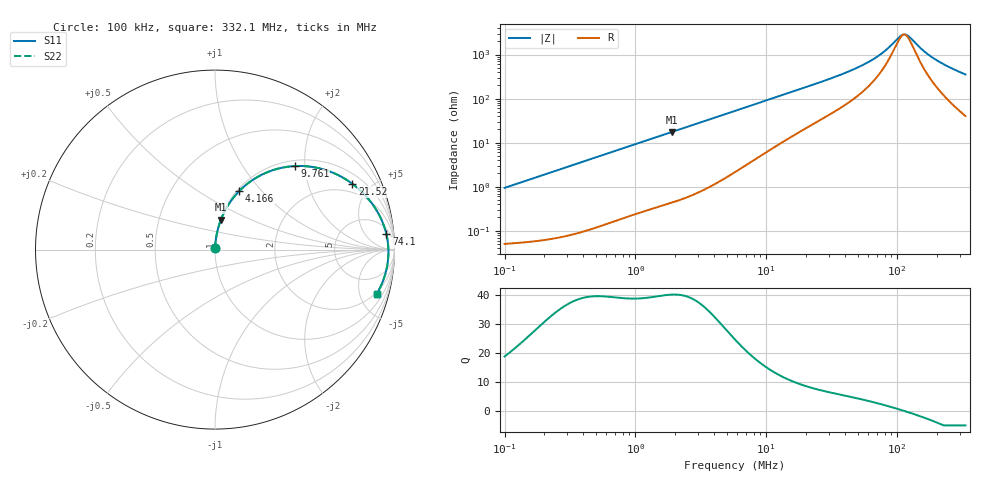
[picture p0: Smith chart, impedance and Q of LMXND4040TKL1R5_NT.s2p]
! LMXND4040TKL1R5_NT  S-PARAMETER MODEL  ( Standard Model )
! Model Generated by TAIYO YUDEN Corporation (https://www.yuden.co.jp/en/)
! Version 1.0
! TAIYO YUDEN Control No. 20251120
! Copyright(c) 2025 TAIYO YUDEN CO.,LTD. All Rights Reserved.
! Product Description (link to TY-COMPAS)
! https://ds.yuden.co.jp/TYCOMPAS/or/detail?pn=LMXND4040TKL1R5NNT&u=M
! Products Name : Inductors
! Characteristics :
!  Inductance : 1.5 [uH] , SRF(min) : 75 [MHz] , DC Resistance(max) : 0.045 [Ohm]
!  Rated Current : Saturation  3300 [mA] , Temp Rise  3100 [mA] (40 [degC])
!  Case Size : 4.0 x 4.0 / 0.157 x 0.157 [mm/inch] , Thickness : 1.8 / 0.071 [mm/inch]
!  (Conditions: Temperature = 25 [degC] , DC Bias Current = 0 [A])
! External Node Assignments :
!  1  o---GGG---o  2
! GND o---------o GND
! Frequency Range : 0.1MHz  -  332.076389MHz  [ 402 STEP ]
# MHz S RI R 50
! Freq[MHz].  S11 Real  S11 Imag  S21 Real  S21 Imag  S12 Real  S12 Imag  S22 Real  S22 Imag
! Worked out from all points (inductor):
!   401 points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, 100 kHz to 332.1 MHz, reference 50 ohm
!   read as one part in series: L = 1.49 uH near 104.1 kHz
!   highest Q = 40 at 1.89 MHz (marker M1), where L = 1.45 uH
!   self-resonance near 113 MHz
!   S11 on the Smith chart (normalised r, x): 100 kHz: 1.00, +0.02; 4.166 MHz: 1.02, +0.76; 9.761 MHz: 1.12, +1.77; 21.52 MHz: 1.48, +3.88; 74.1 MHz: 9, +18; 332.1 MHz: 1.80, -7.02
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0.1  0.00059 0.00939  0.9994 -0.00939  0.9994 -0.00939  0.00059 0.00939
0.388873  0.00224 0.0361  0.9978 -0.0361  0.9978 -0.0361  0.00224 0.0361
1.512219  0.0221 0.1349  0.9779 -0.1349  0.9779 -0.1349  0.0221 0.1349
1.889943  0.0329 0.1662  0.9671 -0.1662  0.9671 -0.1662  0.0329 0.1662
4.166482  0.1339 0.325  0.8661 -0.325  0.8661 -0.325  0.1339 0.325
5.762607  0.2257 0.3981  0.7743 -0.3981  0.7743 -0.3981  0.2257 0.3981
9.761116  0.4449 0.4654  0.5551 -0.4654  0.5551 -0.4654  0.4449 0.4654
14.05902  0.6102 0.4451  0.3898 -0.4451  0.3898 -0.4451  0.6102 0.4451
21.51891  0.766 0.3661  0.234 -0.3661  0.234 -0.3661  0.766 0.3661
22.4092  0.7779 0.357  0.2221 -0.357  0.2221 -0.357  0.7779 0.357
45.55486  0.9162 0.1902  0.0838 -0.1902  0.0838 -0.1902  0.9162 0.1902
59.28911  0.9415 0.1321  0.0585 -0.1321  0.0585 -0.1321  0.9415 0.1321
74.09842  0.9552 0.0852  0.0448 -0.0852  0.0448 -0.0852  0.9552 0.0852
87.14324  0.9615 0.0521  0.0385 -0.0521  0.0385 -0.0521  0.9615 0.0521
106.7246  0.9657 0.0115  0.0343 -0.0115  0.0343 -0.0115  0.9657 0.0115
113.4159  0.9662 -0.00073  0.0338 0.00073  0.0338 0.00073  0.9662 -0.00073
118.1082  0.9663 -0.00888  0.0337 0.00888  0.0337 0.00888  0.9663 -0.00888
125.5132  0.9662 -0.0211  0.0338 0.0211  0.0338 0.0211  0.9662 -0.0211
156.8641  0.9629 -0.0671  0.0371 0.0671  0.0371 0.0671  0.9629 -0.0671
188.2571  0.9562 -0.1065  0.0438 0.1065  0.0438 0.1065  0.9562 -0.1065
245.0144  0.9385 -0.1678  0.0615 0.1678  0.0615 0.1678  0.9385 -0.1678
332.0764  0.9019 -0.2456  0.0981 0.2456  0.0981 0.2456  0.9019 -0.2456
